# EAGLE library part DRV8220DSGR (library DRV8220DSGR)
DRV8220DSGR Source: Datasheet
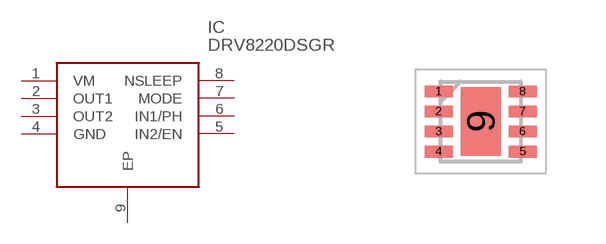
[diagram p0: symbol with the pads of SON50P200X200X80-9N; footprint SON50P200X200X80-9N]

Designator prefix IC

## DRV8220DSGR (DESCRIPTION: DRV8220DSGR; HEIGHT: 0.8mm; MANUFACTURER_NAME: Texas Instruments; MANUFACTURER_PART_NUMBER: DRV8220DSGR)  [SON50P200X200X80-9N]
1  VM  pwr
2  OUT1  pas
3  OUT2  pas
4  GND  pwr
5  IN2/EN  in
6  IN1/PH  in
7  MODE  in
8  NSLEEP  in
9  EP  pwr

## Footprint SON50P200X200X80-9N (pad centres in mm)
DSG
smd 0.7 x 0.3: 1 -1.05,0.75; 2 -1.05,0.25; 3 -1.05,-0.25; 4 -1.05,-0.75; 5 1.05,-0.75; 6 1.05,-0.25; 7 1.05,0.25; 8 1.05,0.75
smd 1 x 1.7: 9 0,0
